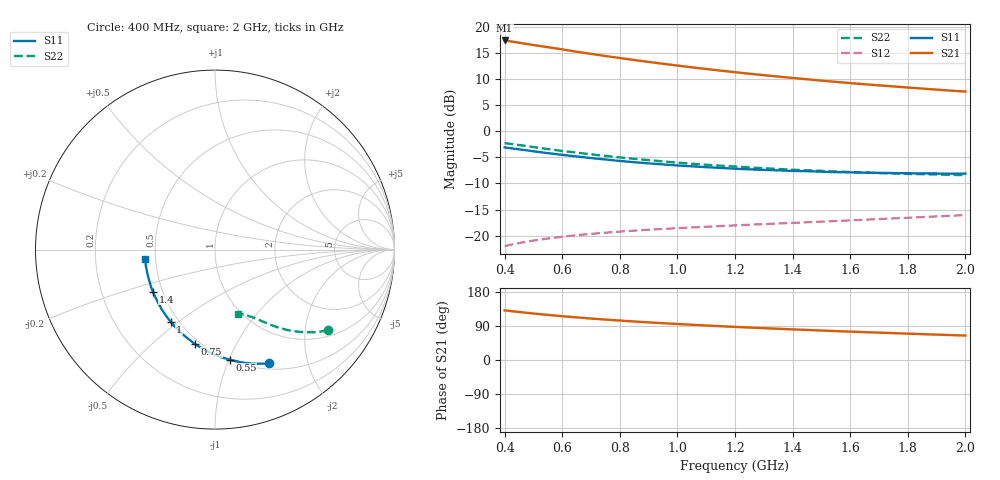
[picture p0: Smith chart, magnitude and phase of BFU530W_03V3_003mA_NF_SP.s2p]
! Filename:  P:\Prog\Test\Noise\ATS_data\Testdata_Net\06 Compressed Noise after Statistics\BFU530W_APM2013_09_A05_03p3V_003mA_NF_CM01_D.sf
! Date/Time: Tue 26/Mar/2013 18:06:07
! BFU530W_APM2013_09_A05_03p3V_1to25mA_NF_CM01_Bias3_R.sf
! Noise Parameter Data File
! BFU530W_APM2013_09_A05_03p3V_1to25mA_NF_CM01
! Date/time: Thu Mar 21 19:18:02 2013
! VAR V_out= 3.300000
! VAR I_out= 3.000000
! VAR V_in= 0.810100
! VAR I_in= 0.031610
! Device data file deembeded for feedlines and parallel
! Original file: \06 Compressed Noise after Statistics\BFU530W_APM2013_09_A05_03p3V_003mA_NF_CM01_R.sf
! Feed-files: PR019V01_070313_Feed1.s2p, PR019V01_070313_Feed2.s2p
! Parallel-file: PR019V01_070313_Par.s2p
# MHz S MA R 50
!  Freq-MHz  S11-mag  S11-arg  S21-mag  S21-arg  S12-mag  S12-arg  S22-mag  S22-arg
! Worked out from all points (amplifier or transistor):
!   37 points, 400 MHz to 2 GHz, reference 50 ohm
!   highest |S21| = 17.5 dB at 400 MHz (marker M1)
!   |S21| within 3 dB of that: start of sweep to 751.6 MHz
!   unconditionally stable (mu >= 1): nowhere
!   at 500 MHz: K = 0.36, MSG = 18.8 dB, |S12| = -21.0 dB
!   at 1.1 GHz: K = 0.71, MSG = 15.1 dB, |S12| = -18.3 dB
!   at 2 GHz: K = 0.99, MSG = 11.9 dB, |S12| = -16.1 dB
!   lowest NFmin = 0.52 dB at 420 MHz
!   S11 on the Smith chart (normalised r, x): 400 MHz: 0.57, -1.43; 550 MHz: 0.51, -1.00; 750 MHz: 0.47, -0.70; 1 GHz: 0.45, -0.47; 1.4 GHz: 0.44, -0.25; 2 GHz: 0.44, -0.05
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400  0.7026 -64.5  7.467 131.1  0.07911 57.2  0.7726 -35.5
420  0.6898 -67.1  7.328 129.2  0.08151 56.3  0.7592 -36.6
440  0.6785 -69.7  7.179 127.6  0.08371 55.3  0.7459 -37.7
480  0.6563 -74.5  6.881 124.3  0.08769 53.6  0.7205 -39.7
500  0.6447 -76.9  6.753 122.7  0.08954 52.9  0.7073 -40.6
550  0.6183 -82.5  6.435 119.0  0.0936 51.2  0.6769 -42.8
600  0.5959 -87.9  6.13 115.5  0.09747 49.8  0.6493 -44.7
650  0.5747 -92.7  5.819 112.5  0.1009 48.6  0.6262 -46.4
700  0.5543 -97.6  5.557 109.4  0.1038 47.6  0.6026 -48.1
750  0.5378 -102.0  5.293 106.7  0.1066 46.8  0.5816 -49.3
800  0.5206 -106.3  5.064 104.1  0.1091 46.2  0.5634 -50.7
850  0.5062 -110.5  4.846 101.6  0.1115 45.6  0.5452 -51.8
950  0.4822 -118.0  4.462 97.1  0.1157 44.9  0.5152 -54.0
1000  0.4713 -121.7  4.287 95.0  0.1178 44.7  0.5014 -54.8
1100  0.4536 -128.3  3.973 91.0  0.1215 44.5  0.4785 -56.7
1200  0.4387 -134.6  3.703 87.4  0.1252 44.6  0.4599 -58.3
1300  0.4269 -140.4  3.466 84.0  0.1288 44.8  0.4429 -59.7
1400  0.4176 -145.9  3.26 80.8  0.1324 45.2  0.4286 -61.2
1500  0.4103 -150.9  3.075 77.8  0.1362 45.7  0.418 -62.8
1600  0.4046 -155.8  2.911 74.9  0.1399 46.3  0.4079 -64.1
1750  0.3982 -162.4  2.703 70.9  0.1462 47.4  0.3951 -66.2
2000  0.3935 -172.7  2.411 64.5  0.1574 49.0  0.3807 -70.0
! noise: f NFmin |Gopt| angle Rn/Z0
400  0.5427  0.3521  27.98  0.1352
460  0.5606  0.3411  32.89  0.1338
600  0.576  0.3421  40.66  0.1375
800  0.6229  0.3304  54.51  0.1264
1000  0.6782  0.3308  68.78  0.1205
1200  0.7131  0.3324  83.22  0.1111
1400  0.7319  0.3305  96.56  0.1026
1600  0.744  0.3355  111.3  0.0823
1800  0.8094  0.3545  127.3  0.0732
2000  0.8635  0.3622  143.3  0.0623
